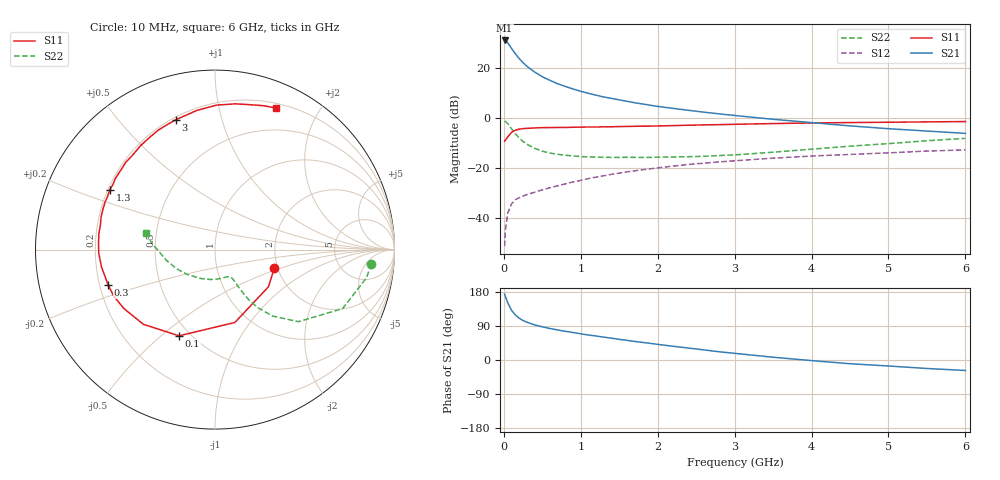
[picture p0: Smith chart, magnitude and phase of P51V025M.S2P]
! SIEMENS Small Signal Semiconductors
! BFP183
! Si NPN RF Bipolar Junction Transistor in SOT143
! VCE = 1 V  IC = 25 mA
! Common Emitter S-Parameters:  March  1996
# GHz  S  MA  R  50
!  f  S11  S21  S12  S22
! GHz  MAG  ANG  MAG  ANG  MAG  ANG  MAG  ANG
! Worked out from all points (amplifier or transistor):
!   36 points, 10 MHz to 6 GHz, reference 50 ohm
!   highest |S21| = 31.2 dB at 10 MHz (marker M1)
!   |S21| within 3 dB of that: start of sweep to 95.6 MHz
!   unconditionally stable (mu >= 1): start of sweep to 10.53 MHz; 417.6 MHz to end of sweep
!   at 250 MHz: K = 0.73, MSG = 26.8 dB, |S12| = -31.2 dB
!   at 1.4 GHz: K = 1.42, MAG = 11.4 dB, |S12| = -22.5 dB
!   at 6 GHz: K = 1.15, MAG = 1.0 dB, |S12| = -12.7 dB
!   S11 on the Smith chart (normalised r, x): 10 MHz: 1.91, -0.46; 100 MHz: 0.44, -0.58; 300 MHz: 0.24, -0.15; 1.3 GHz: 0.21, +0.25; 3 GHz: 0.21, +0.72; 6 GHz: 0.25, +1.49
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0.01  0.3461 -17.6  36.51 174.0  0.0027 83.4  0.8741 -5.2
0.02  0.3627 -34.8  36.09 168.0  0.0056 78.5  0.8591 -10.5
0.05  0.4207 -74.7  32.78 151.0  0.0124 69.4  0.7833 -24.8
0.1  0.5203 -112.6  25.26 131.1  0.0191 52.2  0.6146 -40.8
0.15  0.5764 -133.7  19.72 118.6  0.0232 47.3  0.4884 -49.2
0.2  0.6043 -147.0  15.78 110.2  0.0254 44.6  0.4014 -53.6
0.25  0.6208 -155.3  13.04 104.1  0.0274 43.6  0.3415 -55.9
0.3  0.6268 -161.7  11.1 99.8  0.0293 44.4  0.3007 -56.9
0.4  0.6396 -171.2  8.489 92.7  0.0327 46.3  0.2492 -57.8
0.5  0.6481 -178.2  6.82 87.5  0.0365 48.0  0.2186 -58.1
0.6  0.6501 176.7  5.772 83.1  0.0402 50.1  0.2001 -58.5
0.7  0.6531 172.1  4.934 79.2  0.0441 51.8  0.189 -58.9
0.8  0.6531 167.8  4.353 75.7  0.0482 52.2  0.1807 -59.7
1.1  0.6671 156.7  3.166 65.9  0.0615 54.1  0.1671 -64.4
1.3  0.6736 150.5  2.68 60.3  0.0701 53.7  0.1647 -68.7
1.7  0.6889 138.4  2.051 49.1  0.088 51.9  0.164 -78.2
2.2  0.7125 125.5  1.58 36.2  0.1095 48.1  0.1666 -93.9
3  0.7556 106.8  1.138 17.6  0.1401 40.4  0.1836 -122.0
3.5  0.7825 97.3  0.953 7.3  0.158 35.7  0.2083 -138.6
4.5  0.8201 82.0  0.703 -9.8  0.1878 25.8  0.2754 -166.9
5.5  0.8463 71.3  0.554 -22.4  0.2194 17.2  0.3538 174.2
6  0.8583 66.8  0.497 -27.6  0.2316 12.1  0.3944 166.1
